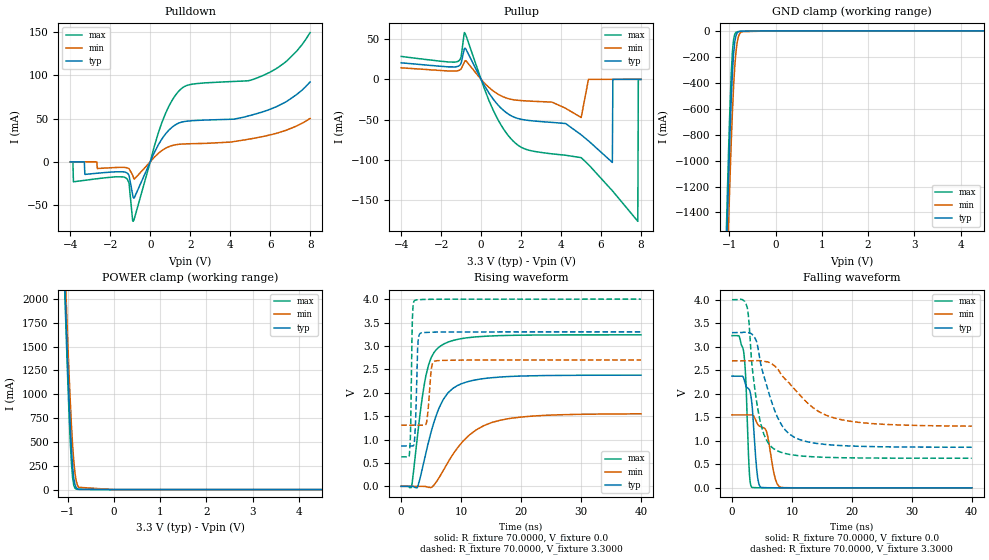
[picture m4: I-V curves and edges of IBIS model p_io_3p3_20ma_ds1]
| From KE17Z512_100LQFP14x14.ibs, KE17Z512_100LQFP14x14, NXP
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[Model] p_io_3p3_20ma_ds1
|   Model p_io_3p3_20ma_ds1
| This model was characterised for following simulation conditions:
| External (pad) voltage:
|   - Typ: 3.3V,   - Min: 2.7V,   - Max: 4.0V
| Library cells for typ/min/max conditions are connected as defined below:
|  pad - External Pad
|  ipp_do_lv - Core Input
|  ipp_obe_lv - Output Buffer Enable
|  abt_close_nor_rst_mv - vdde
|  dvdd - dvdd
|  dvss - dvss
|  esd_boost - vdde
|  ipp_dse_lv - dvdd
|  ipp_ina_280_mv - NC
|  ipp_ina_40_a_mv - NC
|  ipp_ina_40_b_mv - NC
|  ipp_ina_40_c_mv - NC
|  ipp_ina_40_d_mv - NC
|  ipp_ina_40_e_mv - NC
|  ipp_ina_40_f_mv - NC
|  ipp_ina_40_g_mv - NC
|  ipp_ina_40_h_mv - NC
|  ipp_ind_lv - NC
|  vdde - vdde
|  vsse - vsse
| All other pins connected to ground
Model_type I/O
Polarity   Non-Inverting
Enable   Active-High
Vinl =   0.9900V
Vinh =   2.3100V
Vmeas =  1.6500V
Cref =   50.0000F
C_comp   2.8325pF   2.6979pF   3.0285pF
[Model Spec]
| variable   typ   min   max
Vinh   2.3100V   1.8900V   2.8000V
Vinl   0.9900V   0.8100V   1.2000V
S_overshoot_high   3.6000V   3.0000V   4.3000V
S_overshoot_low   -0.3000V   -0.3000V   -0.3000V
Vmeas   1.6500V   1.3500V   2.0000V
[Temperature Range]   25.0000   0.1250k   -40.0000
[Voltage Range]   3.3000V   2.7000V   4.0000V
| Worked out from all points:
|   slope of the pulldown table from 0 to 0.495 V, typ, clamps not added: 21.4 ohm
|   slope of the pullup table from 0 to 0.495 V, typ, clamps not added: 24 ohm
|   rising waveform, R_fixture 70.0000, V_fixture 0.0: 20-80 % time 3.57ns typ, 6.09ns min, 2.21ns max; typ from 0 V to 2.38 V
|   rising waveform, R_fixture 70.0000, V_fixture 3.3000: 20-80 % time 306ps typ, 505ps min, 234ps max; typ from 0.862 V to 3.3 V
|   falling waveform, R_fixture 70.0000, V_fixture 0.0: 20-80 % time 840ps typ, 1.4ns min, 596ps max; typ from 2.38 V to 0 V
|   falling waveform, R_fixture 70.0000, V_fixture 3.3000: 20-80 % time 3.67ns typ, 6.84ns min, 1.98ns max; typ from 3.3 V to 0.863 V
[Pulldown]
|Voltage   I(typ)   I(min)   I(max)
-4V       20uA       20uA       -160uA
-3.87V    20uA       20uA       -190uA
-3.844V   10uA       20uA       -22.99mA
-3.298V   -30uA      10uA       -21.31mA
-3.272V   -14.45mA   20uA       -21.24mA
-1.192V   -12.41mA   -6.69mA    -18.96mA
-1.062V   -15.34mA   -7.788mA   -24.33mA
-854mV    -40.74mA   -17.17mA   -68.52mA
550mV     25.23mA    12.5mA     43.26mA
1.434V    44.79mA    20.25mA    81.67mA
5.568V    57.3mA     28.9mA     98.8mA
8V        92.1mA     50.1mA     149.1mA
[Pullup]
|Voltage   I(typ)   I(min)   I(max)
-4V       20.6mA     14.3mA     28.5mA
-1.152V   16.19mA    10.78mA    22.38mA
-814mV    38.76mA    22.46mA    57.78mA
408mV     -17.55mA   -10.38mA   -27.11mA
1.526V    -45.53mA   -24.96mA   -74.66mA
5.01V     -68.96mA   -47.46mA   -97.36mA
5.374V    -76.5mA    0A         -106mA
6.57V     -103.3mA   20uA       -138.5mA
6.596V    -30uA      20uA       -139.2mA
7.844V    30uA       10uA       -176.5mA
7.87V     30uA       20uA       -190uA
8V        30uA       10uA       -160uA
[GND_clamp]
|Voltage   I(typ)   I(min)   I(max)
-4V       -49.59A    -49.54A    -49.68A
-1.062V   -1.74A     -2.082A    -1.538A
-1.036V   -1.402A    -1.75A     -1.192A
-1.01V    -1.083A    -1.435A    -869.2mA
-984mV    -791.3mA   -1.14A     -579.3mA
-958mV    -535mA     -869mA     -338.2mA
-932mV    -326.2mA   -629.6mA   -164.5mA
-906mV    -175.2mA   -428.2mA   -66.24mA
-880mV    -83.05mA   -270.6mA   -25.06mA
-828mV    -16.12mA   -86.77mA   -7.14mA
-724mV    -2.673mA   -6.605mA   -3.909mA
8V        0A         0A         0A
[POWER_clamp]
|Voltage   I(typ)   I(min)   I(max)
-4V       52.67A     52.45A     52.88A
-1.074V   2.381A     2.6A       2.272A
-1.048V   2.004A     2.236A     1.882A
-1.022V   1.639A     1.885A     1.505A
-970mV    970.2mA    1.235A     814mA
-918mV    434.5mA    688.7mA    285.8mA
-892mV    245.5mA    470.7mA    127mA
-866mV    120.4mA    298.4mA    45.78mA
-814mV    21.03mA    94.6mA     5.402mA
-762mV    3.719mA    24.12mA    1.768mA
0V        97.57pA    2.637nA    84.84pA
8V        0A         0A         0A
[Ramp]
| variable   typ   min   max
dV/dt_r  1.4251/3.5671n   0.9293/6.0875n   1.9421/2.2102n
dV/dt_f  1.4621/3.6710n   0.8326/6.8367n   2.0223/1.9822n
R_load = 70.0000
[Rising Waveform]
R_fixture= 70.0000
V_fixture= 0.0
V_fixture_min= 0.0
V_fixture_max= 0.0
|time   V(typ)   V(min)   V(max)
0s        46.98pV    14.28nV    173.3pV
1.741ns   170.4uV    5.795uV    -6.358mV
2.75ns    -8.126mV   5.272uV    1.107V
4.105ns   699.4mV    -4.763mV   2.351V
4.972ns   1.148V     -25.75mV   2.741V
6.578ns   1.74V      238.3mV    2.999V
7.78ns    1.993V     506.3mV    3.079V
10.3ns    2.203V     961.2mV    3.161V
15.14ns   2.321V     1.365V     3.214V
40ns      2.375V     1.549V     3.237V
[Rising Waveform]
R_fixture= 70.0000
V_fixture= 3.3000
V_fixture_min= 2.7000
V_fixture_max= 4.0000
|time   V(typ)   V(min)   V(max)
0s        862.3mV    1.307V     629.3mV
1.388ns   862.5mV    1.307V     694.6mV
1.591ns   862.6mV    1.307V     1.291V
1.887ns   862.4mV    1.307V     3.615V
2.257ns   1.033V     1.307V     3.972V
2.789ns   3.04V      1.307V     3.986V
3.268ns   3.274V     1.308V     3.991V
4.269ns   3.29V      1.386V     3.995V
5.683ns   3.296V     2.678V     3.997V
40ns      3.3V       2.7V       4V
[Falling Waveform]
R_fixture= 70.0000
V_fixture= 0.0
V_fixture_min= 0.0
V_fixture_max= 0.0
|time   V(typ)   V(min)   V(max)
0s        2.375V     1.551V     3.237V
1.97ns    2.325V     1.551V     2.877V
2.315ns   2.171V     1.551V     2.292V
2.923ns   2.08V      1.552V     272.1mV
3.326ns   1.789V     1.552V     11.11mV
4.197ns   301.4mV    1.372V     3.003mV
4.885ns   10.61mV    1.295V     1.722mV
5.809ns   3.352mV    1.178V     1.038mV
8.179ns   927.1uV    11.47mV    437.7uV
40ns      2.62uV     9.127uV    4.318uV
[Falling Waveform]
R_fixture= 70.0000
V_fixture= 3.3000
V_fixture_min= 2.7000
V_fixture_max= 4.0000
|time   V(typ)   V(min)   V(max)
0s        3.3V       2.7V       4V
2.54ns    3.305V     2.7V       3.838V
2.862ns   3.291V     2.7V       3.484V
3.34ns    3.267V     2.701V     2.595V
4.511ns   2.844V     2.705V     1.532V
5.641ns   2.241V     2.686V     1.042V
7.012ns   1.683V     2.603V     827mV
10.38ns   1.076V     2.106V     695mV
17.08ns   907.2mV    1.485V     643.6mV
40ns      863.2mV    1.312V     629.4mV
